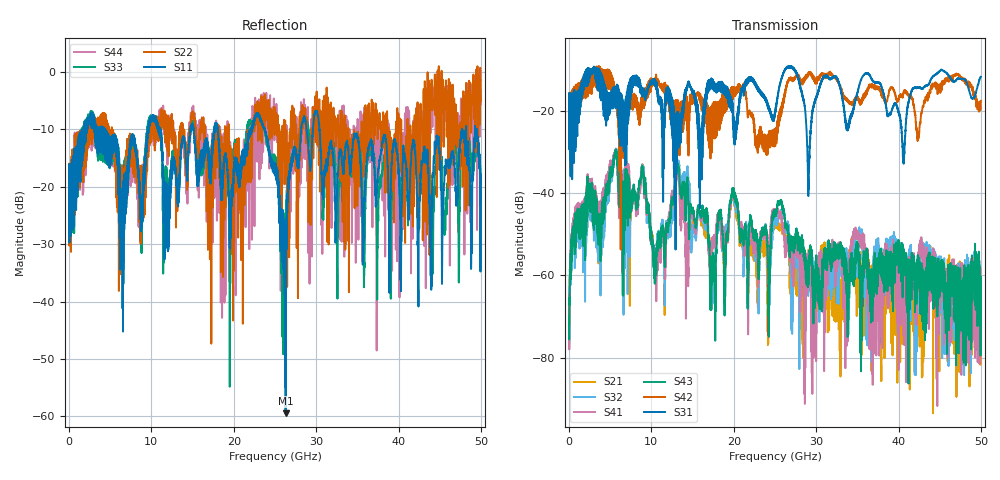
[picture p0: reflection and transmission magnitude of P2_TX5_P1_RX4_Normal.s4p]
!Keysight Technologies,N5225B,MY57041031,A.13.20.10
!Date: Friday, May 31, 2019 11:20:02
!Correction: S11(Full 4 Port(1,2,3,4))
!S12(Full 4 Port(1,2,3,4))
!S13(Full 4 Port(1,2,3,4))
!S14(Full 4 Port(1,2,3,4))
!S21(Full 4 Port(1,2,3,4))
!S22(Full 4 Port(1,2,3,4))
!S23(Full 4 Port(1,2,3,4))
!S24(Full 4 Port(1,2,3,4))
!S31(Full 4 Port(1,2,3,4))
!S32(Full 4 Port(1,2,3,4))
!S33(Full 4 Port(1,2,3,4))
!S34(Full 4 Port(1,2,3,4))
!S41(Full 4 Port(1,2,3,4))
!S42(Full 4 Port(1,2,3,4))
!S43(Full 4 Port(1,2,3,4))
!S44(Full 4 Port(1,2,3,4))
!S4P File: Measurements: <S11,S12,S13,S14>,
!<S21,S22,S23,S24>,
!<S31,S32,S33,S34>,
!<S41,S42,S43,S44>:
# Hz S  dB  R 50.0
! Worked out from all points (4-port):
!   5000 points, 10 MHz to 50 GHz, reference 50 ohm
!   strongest paths, dB at 10 MHz, 12.51 GHz, 25.01 GHz, 37.51 GHz, 50 GHz:
!     S31: -19.5, -17.7, -20.9, -13.2, -11.8
!     S42: -19.4, -19.4, -25.8, -14.5, -17.6
!     S43: -69.9, -42.3, -45.1, -59.2, -60.4
!     S41: -66.6, -40.3, -44.5, -59.5, -70.3
!     S32: -66.7, -45.8, -46.4, -51.4, -66.8
!     S21: -69.0, -43.9, -48.4, -57.2, -63.2
!   lowest |S11| = -59.5 dB at 26.29 GHz (marker M1), VSWR 1.00, Z = 50.1 - j0.016 ohm
!   |S11| at or under -10 dB: 4.282 GHz to 9.568 GHz (5.286 GHz wide, 76.3 % of centre); 23.74 GHz to 28.18 GHz (4.44 GHz wide, 17.1 % of centre); 30.39 GHz to 47.71 GHz (17.32 GHz wide, 44.4 % of centre)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
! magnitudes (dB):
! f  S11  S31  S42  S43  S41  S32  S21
! 10 MHz  -19.8  -19.5  -19.4  -69.9  -66.6  -66.7  -69.0
! 5.61 GHz  -13.3  -17.1  -16.1  -30.0  -29.5  -30.2  -30.0
! 10.56 GHz  -7.8  -14.7  -11.2  -58.2  -62.0  -53.8  -55.5
! 13.09 GHz  -20.6  -28.6  -19.6  -33.3  -34.5  -33.6  -34.8
! 26.29 GHz  -59.5  -9.7  -14.7  -48.4  -54.2  -48.2  -52.9
! 30.01 GHz  -6.8  -16.7  -12.6  -55.1  -69.0  -59.2  -64.1
! 50 GHz  -19.4  -11.8  -17.6  -60.4  -70.3  -66.8  -63.2
